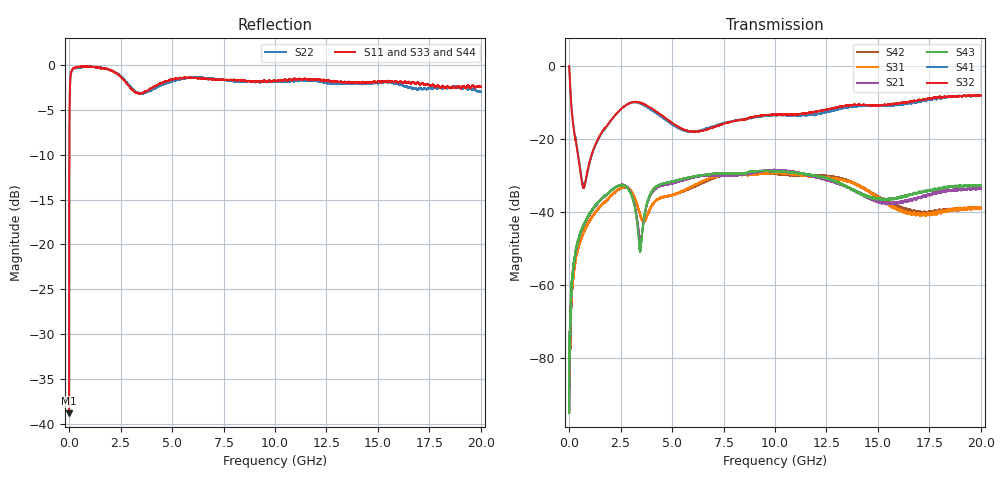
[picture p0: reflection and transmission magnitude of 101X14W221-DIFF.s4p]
!{101X14W221}
!Johanson Technology Inc.
!www.johansontechnology.com
!Test Board Conditions:
!Substrate Type  RO4350B
!Substrate Thickness  10 mil
!Substrate Dk  3.66
!TL Type: GCPW
!TL Trace Width  20 mil
!TL Gap  15 mil
!PART MODE DIFFERENTIAL
!DUT TOPOLOGY	DIFFERENTIAL 4-PORT
!Mounting Pad LxW  20x35 mil
# MHz S  dB  R 50
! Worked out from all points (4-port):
!   20001 points, 300 kHz to 20 GHz, reference 50 ohm
!   strongest paths, dB at 300 kHz, 5 GHz, 10 GHz, 15 GHz, 20 GHz:
!     S32: 0.0, -15.6, -13.3, -10.8, -8.0
!     S41: 0.0, -16.0, -13.5, -10.8, -8.2
!     S43: -79.1, -31.6, -28.8, -36.4, -32.7
!     S21: -76.1, -32.2, -28.5, -37.1, -33.7
!     S31: -75.2, -35.4, -29.3, -36.0, -39.0
!     S42: -80.8, -35.3, -29.5, -35.9, -38.9
!   lowest |S11| = -38.8 dB at 300 kHz (marker M1), VSWR 1.02, Z = 49.9 - j1.14 ohm
!   |S11| at or under -10 dB: start of sweep to 10.96 MHz
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0.3  -38.83 -93.3  -85.67 113.0  -73.14 -91.6  -0.02 -0.6
     -76.09 129.9  -38.67 -101.4  -0.02 -0.4  -79.50 -47.9
     -75.19 -14.1  0.00 -0.3  -38.93 -100.4  -80.30 121.7
     -0.04 -0.5  -80.79 -130.7  -79.14 13.9  -38.61 -89.1
118.298  -0.68 -165.3  -60.45 97.2  -62.28 103.2  -11.35 -67.2
         -60.41 100.1  -0.70 -165.7  -11.73 -67.8  -62.40 110.4
         -62.34 113.0  -11.74 -67.8  -0.62 -165.8  -60.73 103.9
         -11.39 -67.2  -63.60 97.0  -61.16 102.3  -0.63 -165.2
694.29  -0.19 176.9  -43.89 79.6  -45.73 78.8  -32.91 -12.3
        -43.87 80.6  -0.23 174.8  -33.42 -5.7  -45.71 79.5
        -45.85 79.3  -33.34 -5.7  -0.20 174.7  -43.75 79.6
        -32.93 -12.2  -46.01 78.1  -43.67 78.1  -0.20 174.8
2557.262  -1.45 155.6  -32.52 17.2  -33.34 7.5  -11.57 38.2
          -32.58 17.4  -1.35 154.4  -11.61 38.3  -33.40 7.5
          -33.33 7.4  -11.58 38.3  -1.32 154.1  -32.58 18.3
          -11.60 38.3  -33.42 7.4  -32.64 18.2  -1.33 155.2
3450.248  -3.16 160.1  -47.90 -137.9  -40.73 -121.2  -10.29 -1.0
          -47.77 -139.7  -3.17 158.9  -10.00 0.1  -40.81 -119.7
          -40.77 -121.0  -9.99 0.2  -3.05 157.6  -50.73 -147.1
          -10.30 -1.0  -40.91 -119.2  -51.03 -147.6  -2.98 160.6
6189.207  -1.45 150.1  -30.34 35.0  -32.38 34.0  -17.78 -2.6
          -30.34 35.1  -1.39 144.7  -18.02 -9.3  -32.73 32.6
          -32.36 34.2  -17.96 -9.2  -1.47 142.5  -30.07 32.9
          -17.81 -2.7  -32.78 32.3  -30.13 32.5  -1.32 144.5
20000  -2.48 73.6  -33.55 -31.1  -39.00 -86.6  -8.16 -38.7
       -33.67 -30.9  -2.99 67.3  -8.01 -47.1  -38.70 -87.5
       -38.96 -86.3  -7.99 -46.0  -2.74 60.1  -32.66 -36.2
       -8.17 -38.0  -38.91 -88.4  -32.74 -35.9  -2.70 64.2
